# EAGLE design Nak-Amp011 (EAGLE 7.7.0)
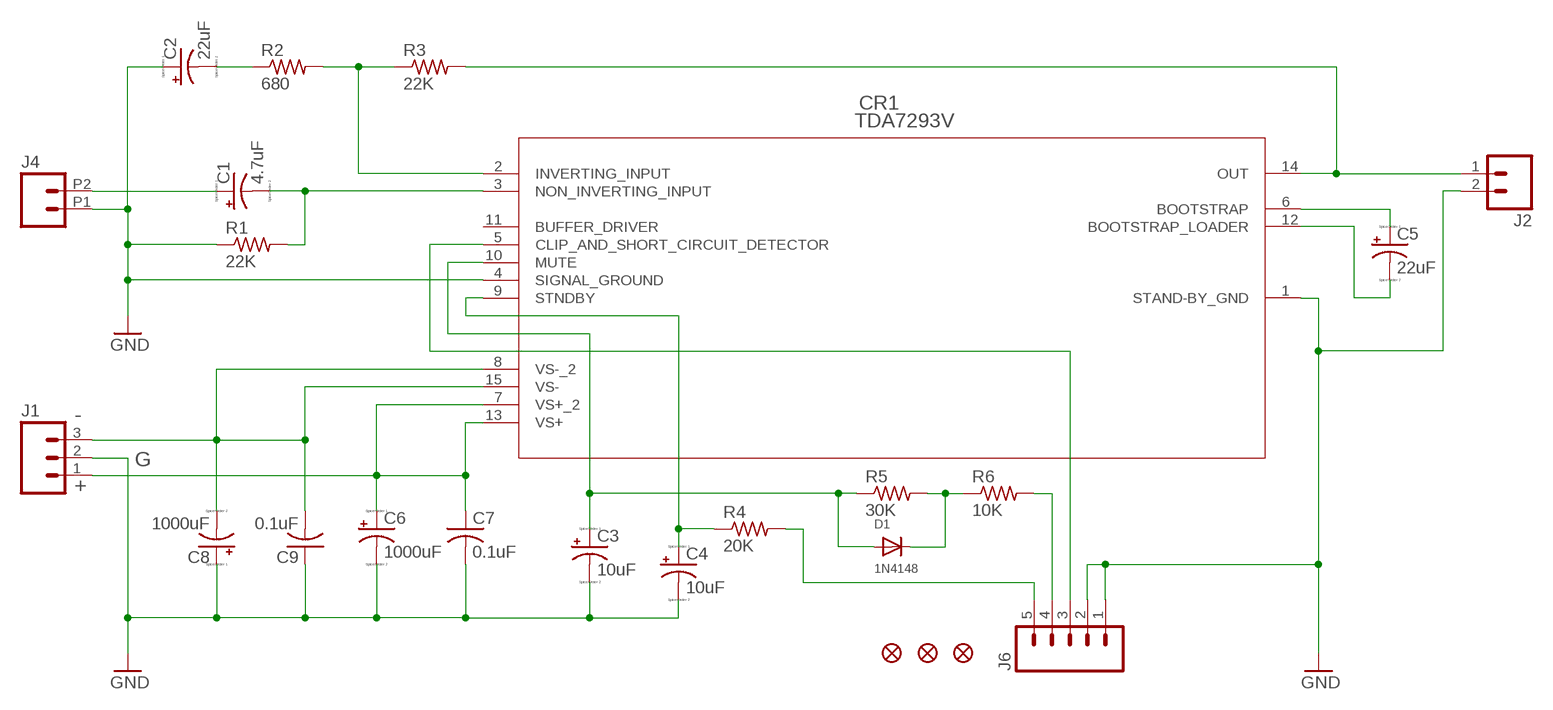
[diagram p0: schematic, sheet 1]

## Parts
C1  4.7uF  CPOL-USE2-5  [E2-5]
C2  22uF  CPOL-USE2.5-7  [E2,5-7]
C3  10uF  CPOL-USE2.5-5  [E2,5-5]
C4  10uF  CPOL-USE2.5-5  [E2,5-5]
C5  22uF  CPOL-USE5-10.5  [E5-10,5]
C6  1000uF  CPOL-USE5-8.5  [E5-8,5]
C7  0.1uF  C-US050-025X075  [C050-025X075]
C8  1000uF  CPOL-USE5-8.5  [E5-8,5]
C9  0.1uF  C-US050-025X075  [C050-025X075]
CR1  TDA7293V  [MULTIWATT15_V]
D1  1N4148  DIODEDO-1N4148  [DO-1N4148]
FD1  FIDUCIAL1X2  [FIDUCIAL-1X2]
FD2  FIDUCIAL1X2  [FIDUCIAL-1X2]
FD3  FIDUCIAL1X2  [FIDUCIAL-1X2]
J1  M03-SCREW-5MM  [SCREWTERMINAL-5MM-3]
J2  M025MM  [SCREWTERMINAL-5MM-2]
J4  M022.54MM_SCREWTERM  [1X02_2.54_SCREWTERM]
J6  M05LOCK  [1X05_LOCK]
R1  22K  R-US_0207/10  [0207/10]
R2  680  R-US_0204/7  [0204/7]
R3  22K  R-US_0204/7  [0204/7]
R4  20K  R-US_0207/7  [0207/7]
R5  30K  R-US_0204/7  [0204/7]
R6  10K  R-US_0207/10  [0207/10]

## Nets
GND: C2.+ C3.- C4.- C6.- C7.2 C8.+ C9.1 CR1.1(STAND-BY_GND) CR1.4(SIGNAL_GROUND) J1.2 J2.2 J4.P1 J6.1 J6.2 R1.1
N$1: C1.- CR1.3(NON_INVERTING_INPUT) R1.2
N$2: C1.+ J4.P2
N$3: J6.5 R4.2
N$4: CR1.2(INVERTING_INPUT) R2.2 R3.1
N$5: J6.4 R6.2
N$6: C2.- R2.1
N$7: CR1.14(OUT) J2.1 R3.2
N$8: C5.+ CR1.6(BOOTSTRAP)
N$9: C5.- CR1.12(BOOTSTRAP_LOADER)
N$10: C6.+ C7.1 CR1.7(VS+_2) CR1.13(VS+) J1.1
N$11: C8.- C9.2 CR1.8(VS-_2) CR1.15(VS-) J1.3
N$12: C4.+ CR1.9(STNDBY) R4.1
N$13: C3.+ CR1.10(MUTE) D1.A R5.1
N$14: D1.C R5.2 R6.1
N$15: CR1.5(CLIP_AND_SHORT_CIRCUIT_DETECTOR) J6.3
Unconnected: CR1.11(BUFFER_DRIVER)

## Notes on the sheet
- -
- G
- +

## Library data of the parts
C1-C6 C8 = resistor:CPOL-US: POLARIZED CAPACITOR, American symbol
C7 C9 = resistor:C-US: CAPACITOR, American symbol
CR1 = STM-TDA7293V:TDA7293V; BUILT_BY: EMA_UL_Team; MANUFACTURER_PART_NUMBER: TDA7293V; VENDOR: STMicroelectronics
D1 = adafruit:DIODE: Diode
FD1-FD3 = SparkFun-Aesthetics:FIDUCIAL: Fiducial Alignment Points
J1 = SparkFun-Connectors:M03: Header 3 Standard 3-pin 0.1" header. Use with straight break away headers (SKU : PRT-00116), right angle break away headers (PRT-00553), swiss pins (PRT-00743), machine pins (PRT-00117), and female headers (PRT-00115). Molex polarized connector foot print use with SKU : PRT-08232 with associated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; STOREFRONT_ID: PRT-08433
J2 = SparkFun-Connectors:M02: Standard 2-pin 0.1" header. Use with; STOREFRONT_ID: PRT-08432
J4 = SparkFun-Connectors:M02: Standard 2-pin 0.1" header. Use with
J6 = SparkFun-Connectors:M05: Header 5 Standard 5-pin 0.1" header. Use with straight break away headers (SKU : PRT-00116), right angle break away headers (PRT-00553), swiss pins (PRT-00743), machine pins (PRT-00117), and female headers (PRT-00115). Molex polarized connector foot print use with SKU : PRT-08230 with associated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
R1-R6 = resistor:R-US_: RESISTOR, American symbol

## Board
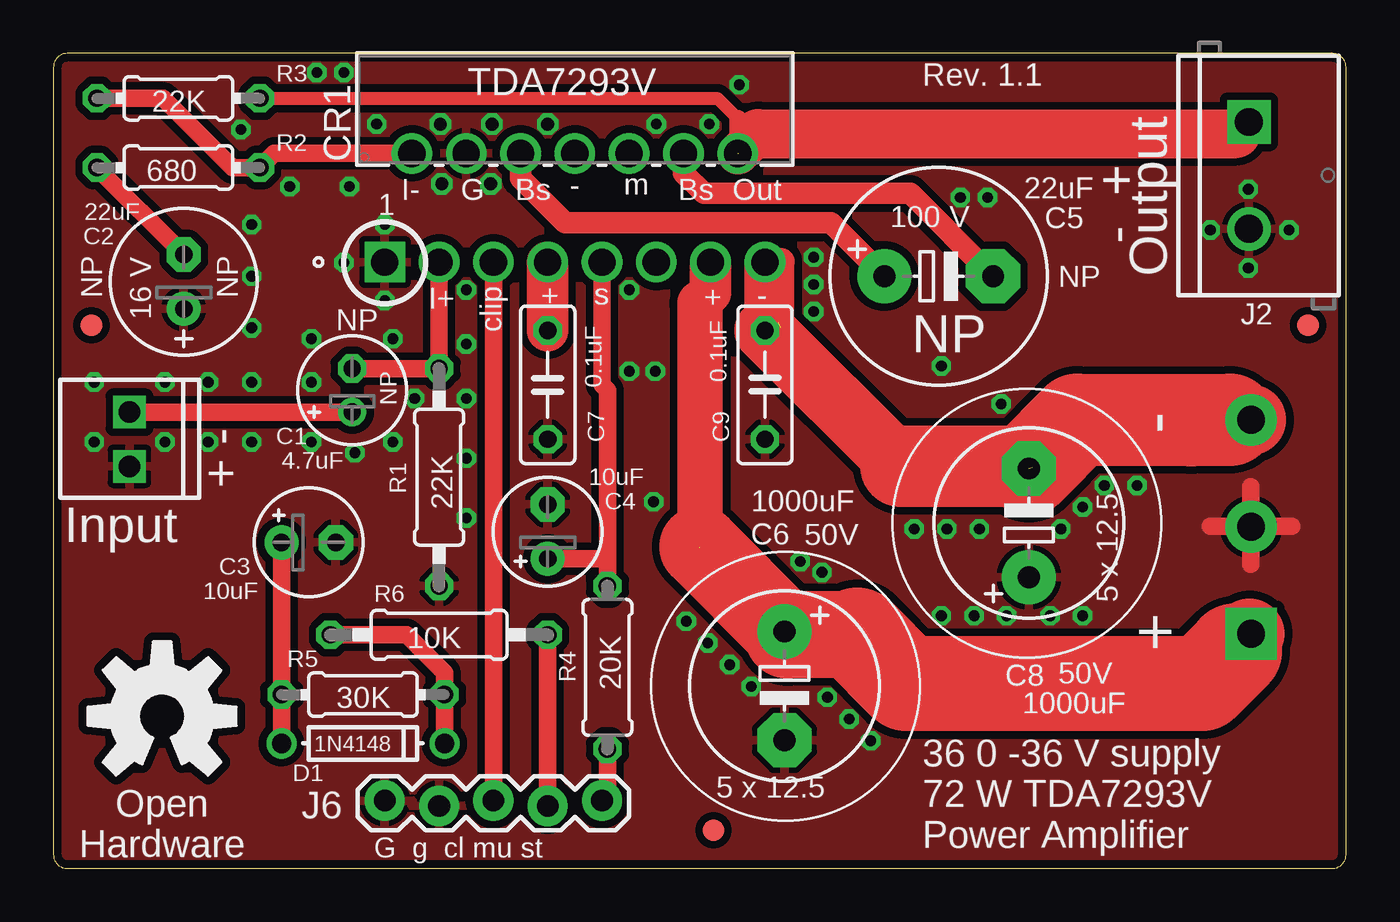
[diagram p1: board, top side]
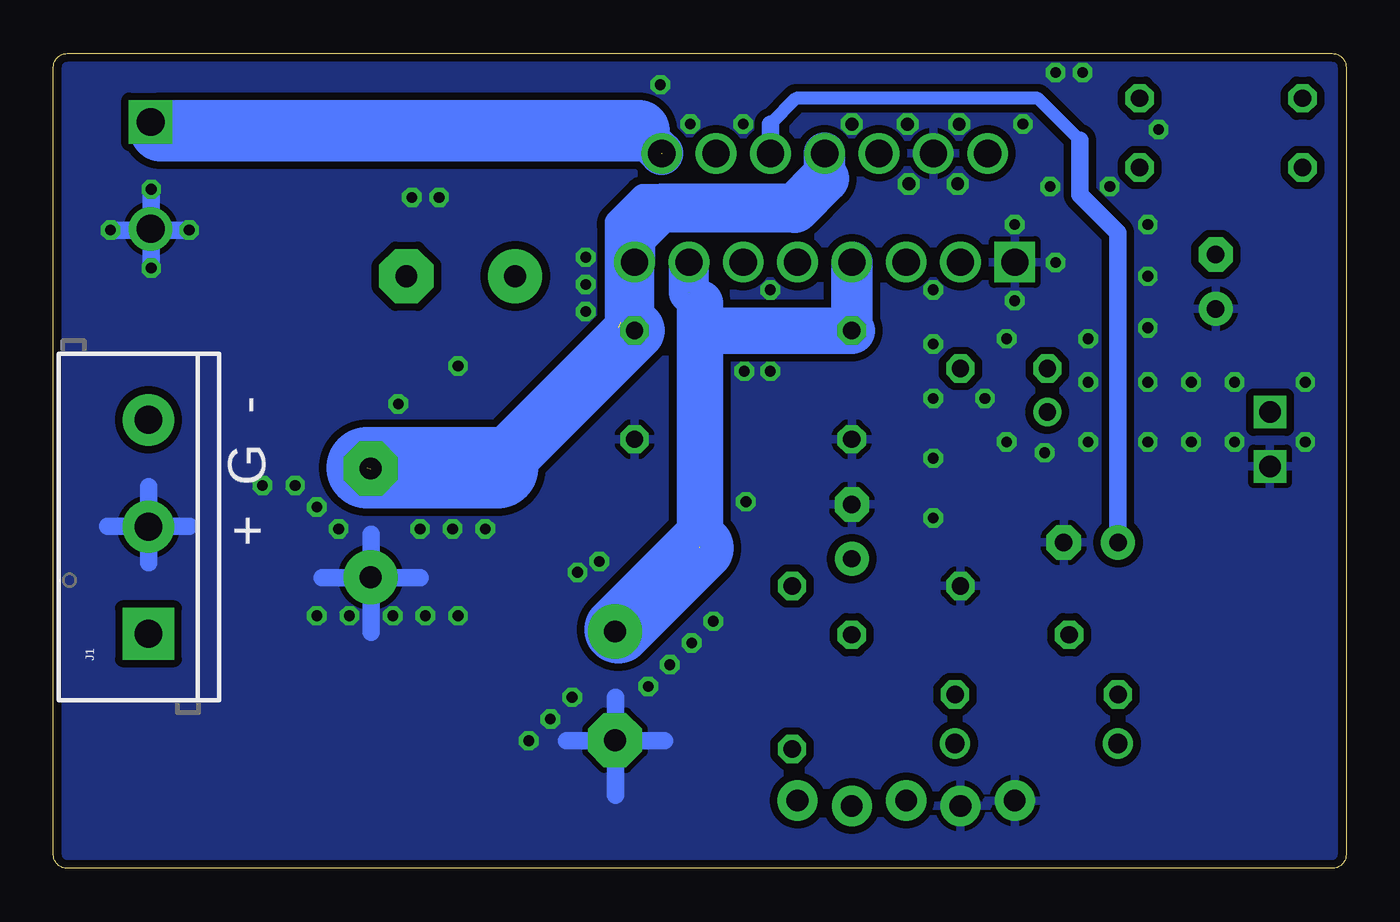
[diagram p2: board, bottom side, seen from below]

Size 60.45 x 38.1 mm. Coordinates in mm from the lower left corner, seen from the top.
Outline: 0,37.47 0,0.64 arc90 0.64,0 59.82,0 arc90 60.45,0.64 60.45,37.47 arc90 59.82,38.1 0.64,38.1 arc90 0,37.47
Copper layers (1*16): Top 0.035mm / dielectric 1.5mm / Bottom 0.035mm
Design rules "default *": minimum track width 8mil, minimum drill 9mil, track to track 14mil, track to pad 14mil, pad to pad 14mil, via to via 14mil, smd to smd 8mil, copper to edge 15mil, drill to drill 9mil, minimum pad ring 10mil, minimum via ring 8mil, stop-mask expansion 4mil, vias tented up to drill 24mil, thermal gap 10mil

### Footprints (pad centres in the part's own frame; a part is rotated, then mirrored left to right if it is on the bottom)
E2-5 = drill 0.813 pad 1.27: + -1.016,0 | drill 0.813 pad 1.27 octagon: - 1.016,0
E2,5-7 = drill 0.813 pad 1.6: + -1.27,0 | drill 0.813 pad 1.6 octagon: - 1.27,0
E2,5-5 = drill 0.813 pad 1.6: + -1.27,0 | drill 0.813 pad 1.6 octagon: - 1.27,0
E5-10,5 = drill 1.016 pad 2.54: + -2.54,0 | drill 1.016 pad 2.54 octagon: - 2.54,0
E5-8,5 = drill 1.016 pad 2.54: + -2.54,0 | drill 1.016 pad 2.54 octagon: - 2.54,0
C050-025X075 = drill 0.813 octagon: 1 -2.54,0; 2 2.54,0
MULTIWATT15_V = drill 1.27 pad 1.778 square: 1 -17.78,-14.326 | drill 1.27 pad 1.778: 2 -16.51,-9.246; 3 -15.24,-14.326; 4 -13.97,-9.246; 5 -12.7,-14.326; 6 -11.43,-9.246; 7 -10.16,-14.326; 8 -8.89,-9.246; 9 -7.62,-14.326; 10 -6.35,-9.246; 11 -5.08,-14.326; 12 -3.81,-9.246; 13 -2.54,-14.326; 14 -1.27,-9.246; 15 0,-14.326
DO-1N4148 = drill 0.9: A -3.81,0; C 3.81,0
FIDUCIAL-1X2 = smd 1 x 1: 1 0,0
SCREWTERMINAL-5MM-3 = drill 1.3 pad 2.413 square: 1 0,0 | drill 1.3 pad 2.413: 2 5,0; 3 10,0
SCREWTERMINAL-5MM-2 = drill 1.3 pad 2.032 square: 1 0,0 | drill 1.3 pad 2.032: 2 5,0
1X02_2.54_SCREWTERM = drill 1.016 square: P1 2.54,0; P2 0,0
1X05_LOCK = drill 1.016 pad 1.88: 1 0,0.127; 2 2.54,-0.127; 3 5.08,0.127; 4 7.62,-0.127; 5 10.16,0.127
0207/10 = drill 0.813 octagon: 1 -5.08,0; 2 5.08,0
0204/7 = drill 0.813 octagon: 1 -3.81,0; 2 3.81,0
0207/7 = drill 0.813 octagon: 1 -3.81,0; 2 3.81,0

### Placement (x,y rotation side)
C1  13.97,22.35 90 top
C2  6.1,27.43 90 top
C3  11.94,15.24 0 top
C4  23.11,15.75 90 top
C5  41.4,27.69 0 top
C6  34.19,8.53 270 top
C7  23.11,22.61 270 top
C8  45.62,16.15 90 top
C9  33.27,22.61 90 top
CR1  33.27,42.67 0 top
D1  14.48,5.84 0 top
FD1  1.78,25.4 0 top
FD2  58.67,25.4 0 top
FD3  30.86,1.78 0 top
J1  56.01,10.97 90 bottom
J2  55.91,34.9 270 top
J4  3.56,21.34 270 top
J6  15.49,3.05 0 top
R1  18.03,18.29 90 top
R2  5.84,32.77 0 top
R3  5.84,36 0 top
R4  25.91,9.4 270 top
R5  14.48,8.13 0 top
R6  18.03,10.92 0 top
U$1  [OSHW-LOGO-L_COPPER]  5.08,7.11 0 top
U$2  [OSHW-LOGO-L]  5.08,7.11 0 top

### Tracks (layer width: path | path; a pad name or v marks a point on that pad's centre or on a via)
GND  (via drill 0.5, 0.6)
  Top 0.813: 56.01,17.84 56.01,14.22 | 54.1,16 57.91,16
  Bottom 0.813: v54.1,29.84 v57.78,29.84 | v55.88,31.75 v55.88,28.07 | 45.59,11.05 45.59,15.62 | 47.88,13.59 43.31,13.59 | 31.88,5.97 36.45,5.97 | 34.16,8 34.16,3.43 | 54.1,16 57.91,16 | 56.01,17.84 56.01,14.29
  other vias: 18.1,34.8 20.51,34.8 18.16,32 20.45,32 15.49,30.1 15.49,26.54 13.59,28.32 19.3,27.05 26.92,23.24 28.14,23.24 35.56,28.57 28.19,34.8 8.76,34.54 9.27,27.69 9.27,25.27 9.27,30.1 11.05,31.88 12.06,22.73 13.84,31.88 12.06,24.77 16.89,21.97 26.92,27.05 12.06,19.94 5.21,22.73 5.21,19.94 7.24,22.73 7.24,19.94 1.91,19.94 1.91,22.73 19.3,24.51 19.3,21.97 19.3,19.18 19.3,16.38 30.67,34.8 42.42,31.37 43.69,31.37 35.56,27.3 23.11,34.8 13.59,37.21 12.32,37.21 15.11,34.8 32.07,36.64 28.07,17.14 29.59,11.56 30.61,10.54 31.62,9.53 32.64,8.51 35.94,13.84 34.92,14.35 41.53,11.81 36.2,8 37.21,6.99 38.23,5.97 44.58,11.81 43.05,11.81 46.61,11.81 48.13,11.81 49.15,17.91 50.67,17.91 48.13,16.89 40.26,15.88 41.78,15.88 43.31,15.88 44.32,21.72 41.53,23.5 47.12,15.88 35.56,26.04 9.27,22.73 9.27,19.94 15.88,19.94 14.1,19.43 15.88,24.77
  pour Bottom: 0,0 60.45,0 60.45,38.1 0,38.1
  pour Top: 0,0 60.45,0 60.45,37.85 0,37.85
N$1
  Top 0.813: CR1.3 R1.2 C1.-
N$2
  Top 0.813: C1.+ J4.P2
N$3
  Top 0.813: J6.5 25.91,3.05 R4.2
N$4
  Top 0.813: CR1.2 10.31,33.43 R2.2 8.38,32.77 5.14,36.01 R3.1
N$5
  Top 0.813: J6.4 R6.2
N$6
  Top 0.813: R2.1 C2.-
N$7  (1 unrouted)
  Top 0.61: R3.2 31.05,36.01 32,35.05
  Top 0.813: 32,35.05 CR1.14
  Top 1.93: 32,33.4 32.96,34.35 | 55.31,34.35 55.88,34.92
  Top 2.286: 32.96,34.35 55.31,34.35
  Bottom 1.93: J2.1 55.85,34.9 55.44,34.48
  Bottom 2.032: 33.06,34.48 CR1.14
  Bottom 2.87: 55.44,34.48 33.06,34.48
N$8
  Top 1.016: CR1.6 21.84,32.26 23.93,30.18 36.37,30.18 C5.+
N$9
  Top 1.016: CR1.12 29.46,32.51 30.42,31.56 40.07,31.56 C5.-
N$10  (2 unrouted)
  Top 1.93: C7.1 CR1.7 | CR1.13 30.73,26.92 30.23,26.42
  Top 2.134: 30.23,26.42 30.23,15.05
  Top 2.54: J1.1 55.93,10.97 | 34.34,10.92 C6.+
  Top 3.302: 55.93,10.97 55.24,10.16
  Top 3.81: C6.+ 30.23,15.05
  Top 4.064: 37.59,10.92 34.34,10.92
  Top 4.445: 55.24,10.16 53.72,8.64 39.88,8.64 37.59,10.92
  Bottom 1.016: 30.73,26.92 30.73,26.16 29.72,25.15
  Bottom 1.88: 30.23,26.42 30.73,26.92 30.73,28.32
  Bottom 1.93: 29.72,25.15 30.23,25.15 | C7.1 CR1.7
  Bottom 2.184: 30.23,15.05 30.23,25.15 30.23,26.42 | C7.1 29.72,25.15
  Bottom 3.175: 30.23,14.99 34.04,11.18
N$11  (2 unrouted)
  Top 1.27: 34.04,25.27 34.04,28.38
  Top 1.93: C9.2 CR1.15
  Top 2.87: C9.2 39.62,18.8
  Top 3.302: J1.3 55.01,20.97
  Top 3.81: 39.62,18.8 45.77,18.8
  Top 4.318: 55.01,20.97 53.21,20.95 47.9,20.97 C8.-
  Bottom 0.406: 32.13,30.86 32.13,31.37 32,31.5 | 33.91,30.1 34.04,30.1 34.16,30.23
  Bottom 1.016: 32,31.5 32.89,31.5 34.16,30.23
  Bottom 1.524: 33.91,30.1 33.91,25.53
  Bottom 1.88: C9.2 33.27,28.32
  Bottom 1.93: CR1.8 24.38,32.26 | 33.27,29.72 CR1.15
  Bottom 2.286: 24.38,32.26 25.78,30.86 32.13,30.86 33.27,29.72
  Bottom 2.794: 39.69,18.73 C9.2
  Bottom 3.81: 45.78,18.73 39.69,18.73
N$12
  Top 0.813: CR1.9 25.65,22.61 25.91,22.35 25.91,14.48 | C4.+ 25.91,14.48 | 25.91,14.48 R4.1
N$13
  Top 0.813: C3.+ R5.1 D1.A
  Bottom 0.61: 12.45,34.04 14.41,36.01 25.72,36.01 26.92,34.8
  Bottom 0.813: C3.+ 10.67,29.72 12.45,31.5 12.45,34.04 | 26.92,34.8 CR1.10
N$14
  Top 0.813: D1.C R5.2 18.29,9.14 16.51,10.92 R6.1
N$15
  Top 0.813: CR1.5 J6.3

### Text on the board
tNames: Rev. 1.1 | 1 | I- | G | Bs | - | m | Bs | Out | 100 V | - + | Output | NP | NP | clip | NP | 16 V | I+ | + | s | + | - | NP | NP | NP | - | + - | Input | 50V | 5 x 12.5 | + | 50V | 5 x 12.5 | Open / Hardware | G g cl mu st | 36 0 -36 V supply / 72 W TDA7293V / Power Amplifier
bNames: + G -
